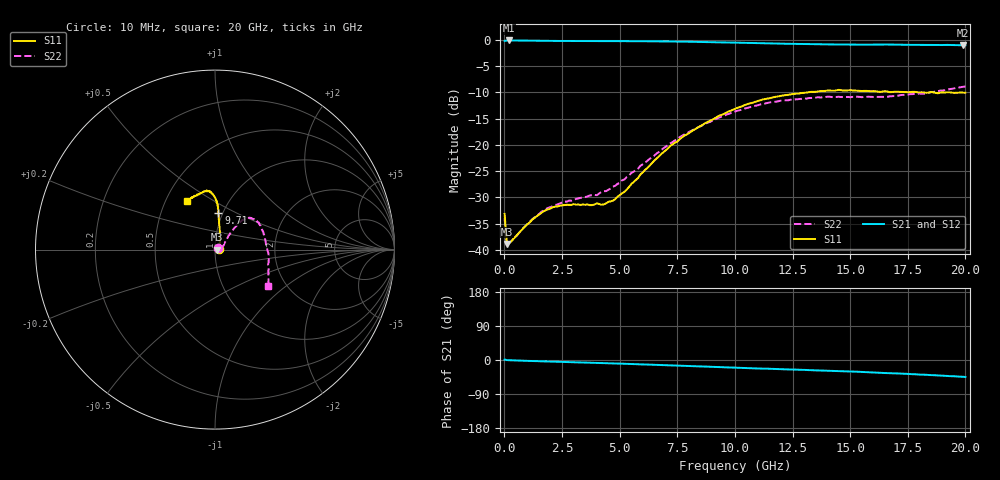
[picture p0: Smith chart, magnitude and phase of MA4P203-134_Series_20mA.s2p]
! AWR Design Environment (9226) Thu Aug 19 14:29:25 2021
! Document = '20mA'
! nPorts: 2, nXvals: 201
# GHz S DB R 50
!Freq DBS11 AngS11 DBS21 AngS21 DBS12 AngS12 DBS22 AngS22
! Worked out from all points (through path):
!   201 points, 10 MHz to 20 GHz, reference 50 ohm
!   highest |S21| = -0.15 dB at 210 MHz (marker M1); lowest = -1.1 dB at 19.91 GHz (marker M2)
!   group delay of S21, straight-line fit = 5.95 ps
!   lowest |S11| = -38.9 dB at 110 MHz (marker M3), VSWR 1.02, Z = 51.1 + j0.0112 ohm
!   |S11| at or under -10 dB: start of sweep to 13.18 GHz; 17.91 GHz to 18.46 GHz (555.2 MHz wide, 3.05 % of centre); 18.58 GHz to end of sweep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
!   |S22| runs from -39.3 to -8.9 dB; largest |S21 - S12| = 0.043
!   S11 on the Smith chart (normalised r, x): 10 MHz: 1.04, +0.01; 9.71 GHz: 0.95, +0.41; 20 GHz: 0.64, +0.38
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0.01  -33.14 11.5  -0.22 1.2  -0.20 0.8  -33.92 29.6
0.11  -38.89 0.6  -0.15 -0.3  -0.14 -0.3  -39.28 1.2
0.21  -38.71 3.0  -0.15 -0.5  -0.14 -0.5  -38.69 5.0
1.21  -34.23 -4.1  -0.20 -2.7  -0.19 -2.6  -34.16 -3.4
1.71  -32.63 -11.7  -0.23 -3.6  -0.21 -3.4  -32.48 -11.0
2.41  -31.57 -18.4  -0.25 -4.8  -0.23 -4.5  -31.14 -16.7
3.41  -31.33 -12.3  -0.26 -6.7  -0.24 -6.1  -29.99 -11.3
4.01  -31.16 0.2  -0.26 -7.8  -0.25 -7.2  -29.59 -1.7
4.31  -31.33 11.1  -0.27 -8.2  -0.25 -7.7  -28.82 3.0
4.71  -30.61 24.2  -0.28 -9.0  -0.26 -8.4  -27.98 10.7
5.21  -28.92 41.8  -0.28 -10.0  -0.26 -9.3  -26.59 20.5
6.71  -22.21 69.3  -0.32 -13.1  -0.29 -12.2  -21.33 41.6
7.81  -18.24 78.1  -0.38 -15.5  -0.37 -14.5  -18.01 46.8
9.71  -13.68 84.8  -0.53 -19.6  -0.52 -18.3  -14.14 48.0
10.01  -13.15 84.9  -0.56 -20.3  -0.55 -18.9  -13.67 48.1
11.21  -11.38 87.7  -0.67 -22.9  -0.67 -21.1  -12.25 45.2
13.41  -9.93 94.3  -0.86 -26.8  -0.82 -25.2  -11.04 35.1
14.51  -9.55 97.8  -0.92 -29.3  -0.86 -27.3  -10.86 27.9
16.71  -9.98 108.5  -0.95 -34.8  -0.87 -32.4  -10.80 3.4
18.21  -10.04 116.7  -1.00 -38.7  -0.90 -37.1  -10.27 -15.5
19.91  -10.09 121.2  -1.07 -44.3  -1.00 -43.1  -8.96 -33.4
20  -10.10 120.0  -1.07 -45.0  -1.01 -43.3  -8.88 -34.3
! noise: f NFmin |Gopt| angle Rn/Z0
0.01  0  1  0  2e-20
2.21  0  1  0  2e-20
4.41  0  1  0  2e-20
6.61  0  1  0  2e-20
8.81  0  1  0  2e-20
11.11  0  1  0  2e-20
13.31  0  1  0  2e-20
15.51  0  1  0  2e-20
17.71  0  1  0  2e-20
20  0  1  0  2e-20
